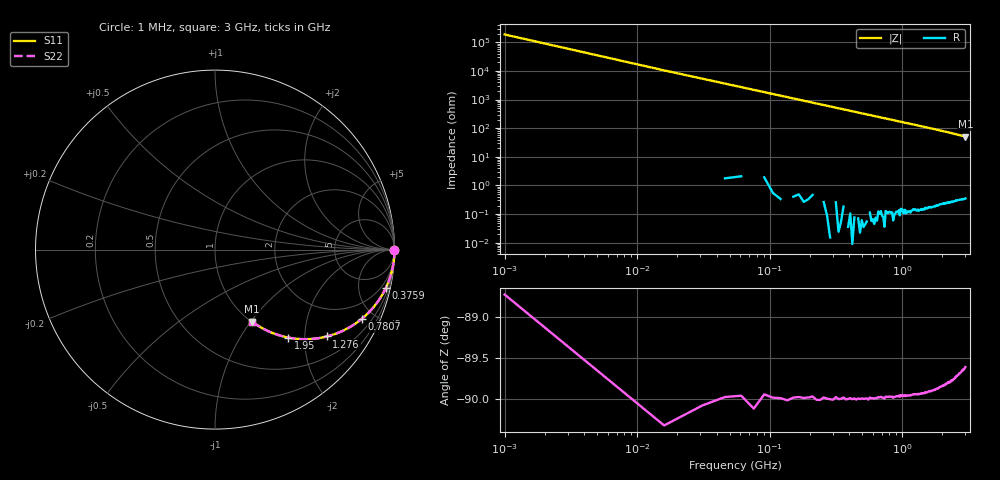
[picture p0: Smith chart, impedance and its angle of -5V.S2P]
!Keysight Technologies,E4991B,MY54301043,A.02.04
!Date: Thu Nov 16 21:16:28 2023
!Data:
!Freq	S11	S21	S12	S22
# Hz S MA R 50
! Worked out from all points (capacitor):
!   201 points, 1 MHz to 3 GHz, reference 50 ohm
!   read as one part in series: C = 959 fF near 15.99 MHz
!   lowest |Z| = 50.9 ohm at 3 GHz (marker M1)
!   S11 on the Smith chart (normalised r, x): 1 MHz: open; 375.9 MHz: 1.00, -8.83; 780.7 MHz: 1.00, -4.23; 1.276 GHz: 1.00, -2.57; 1.95 GHz: 1.00, -1.65; 3 GHz: 1.01, -1.02
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1000000  1 -0.0  0.0005369 88.7  0.0005369 88.7  1 -0.0
1.5995e7  1 -0.6  0.009622 89.8  0.009622 89.8  1 -0.6
3.099e7  0.9999 -1.1  0.01867 89.0  0.01867 89.0  0.9999 -1.1
4.5985e7  0.9996 -1.6  0.0277 88.4  0.0277 88.4  0.9996 -1.6
6.098e7  0.9993 -2.1  0.03667 87.9  0.03667 87.9  0.9993 -2.1
7.5975e7  0.999 -2.6  0.04574 87.5  0.04574 87.5  0.999 -2.6
1.05965e8  0.9979 -3.7  0.0637 86.3  0.0637 86.3  0.9979 -3.7
1.35955e8  0.9967 -4.7  0.08169 85.3  0.08169 85.3  0.9967 -4.7
1.8094e8  0.9941 -6.2  0.1084 83.8  0.1084 83.8  0.9941 -6.2
2.25925e8  0.9909 -7.8  0.1349 82.3  0.1349 82.3  0.9909 -7.8
2.7091e8  0.9869 -9.3  0.1611 80.7  0.1611 80.7  0.9869 -9.3
3.75875e8  0.9753 -12.8  0.221 77.2  0.221 77.2  0.9753 -12.8
5.1083e8  0.9556 -17.1  0.2945 72.9  0.2945 72.9  0.9556 -17.1
6.3079e8  0.9344 -20.9  0.3561 69.1  0.3561 69.1  0.9344 -20.9
7.8074e8  0.9041 -25.3  0.427 64.7  0.427 64.7  0.9041 -25.3
1.005665e9  0.8534 -31.4  0.5205 58.6  0.5205 58.6  0.8534 -31.4
1.275575e9  0.7892 -37.8  0.6133 52.1  0.6133 52.1  0.7892 -37.8
1.5005e9  0.736 -42.5  0.6758 47.4  0.6758 47.4  0.736 -42.5
1.95035e9  0.6366 -50.3  0.7695 39.5  0.7695 39.5  0.6366 -50.3
2.01033e9  0.6243 -51.2  0.7794 38.6  0.7794 38.6  0.6243 -51.2
2.505165e9  0.5312 -57.7  0.8448 32.1  0.8448 32.1  0.5312 -57.7
3e9  0.4524 -62.7  0.8887 26.9  0.8887 26.9  0.4524 -62.7
